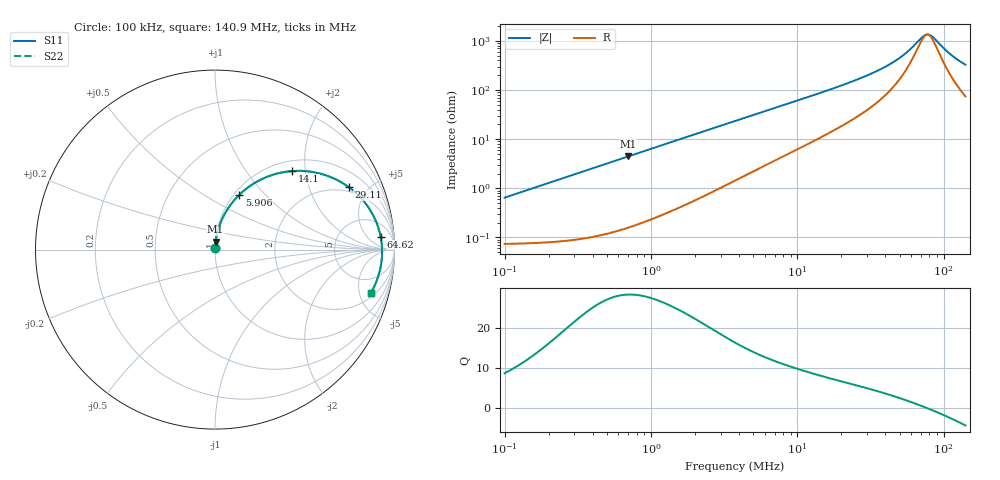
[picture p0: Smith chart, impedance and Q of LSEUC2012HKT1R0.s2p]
! LSEUC2012HKT1R0  S-PARAMETER MODEL  ( Standard Model )
! Model Generated by TAIYO YUDEN Corporation (http://www.ty-top.com)
! Version 1.0
! TAIYO YUDEN Control No. 20230502
! Copyright(c) 2023 TAIYO YUDEN CO.,LTD. All Rights Reserved.
! Product Description (link to TY-COMPAS)
! https://ds.yuden.co.jp/TYCOMPAS/or/detail?pn=LSEUC2012HKT1R0M&u=M
! Products Name : Inductors
! Characteristics :
!  Inductance : 1.0 [uH] , SRF(min) : - [Hz] , DC Resistance(max) : 0.078 [Ohm]
!  Rated Current : Saturation  3200 [mA] , Temp Rise  2300 [mA] (40 [degC])
!  Case Size : 2.0 x 1.2 / 0.079 x 0.047 [mm/inch] , Thickness : 0.8 / 0.031 [mm/inch]
!  (Conditions: Temperature = 25 [degC] , DC Bias Current = 0 [A])
! External Node Assignments :
!  1  o---GGG---o  2
! GND o---------o GND
! Frequency Range : 0.1MHz  -  140.89697MHz  [ 402 STEP ]
# MHz S RI R 50
! Freq[MHz].  S11 Real  S11 Imag  S21 Real  S21 Imag  S12 Real  S12 Imag  S22 Real  S22 Imag
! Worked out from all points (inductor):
!   401 points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, 100 kHz to 140.9 MHz, reference 50 ohm
!   read as one part in series: L = 1.02 uH near 103.7 kHz
!   highest Q = 28.2 at 695.6 kHz (marker M1), where L = 1.02 uH
!   self-resonance near 77.34 MHz
!   S11 on the Smith chart (normalised r, x): 100 kHz: 1.00, +0.01; 5.906 MHz: 1.06, +0.72; 14.1 MHz: 1.21, +1.70; 29.11 MHz: 1.73, +3.73; 64.62 MHz: 13, +13; 140.9 MHz: 2.48, -6.36
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0.1  0.00078 0.0064  0.9992 -0.0064  0.9992 -0.0064  0.00078 0.0064
0.336853  0.0014 0.0215  0.9986 -0.0215  0.9986 -0.0215  0.0014 0.0215
0.695555  0.00353 0.0441  0.9965 -0.0441  0.9965 -0.0441  0.00353 0.0441
1.134703  0.00781 0.0712  0.9922 -0.0712  0.9922 -0.0712  0.00781 0.0712
2.101545  0.0229 0.1283  0.9771 -0.1283  0.9771 -0.1283  0.0229 0.1283
3.753625  0.0636 0.2152  0.9364 -0.2152  0.9364 -0.2152  0.0636 0.2152
5.905507  0.1348 0.3046  0.8652 -0.3046  0.8652 -0.3046  0.1348 0.3046
8.641209  0.2373 0.3806  0.7627 -0.3806  0.7627 -0.3806  0.2373 0.3806
12.64421  0.3832 0.4318  0.6168 -0.4318  0.6168 -0.4318  0.3832 0.4318
14.09696  0.431 0.4377  0.569 -0.4377  0.569 -0.4377  0.431 0.4377
20.25678  0.5955 0.4209  0.4045 -0.4209  0.4045 -0.4209  0.5955 0.4209
29.10821  0.7442 0.3489  0.2558 -0.3489  0.2558 -0.3489  0.7442 0.3489
42.59248  0.8584 0.2297  0.1416 -0.2297  0.1416 -0.2297  0.8584 0.2297
52.94195  0.9001 0.1496  0.0999 -0.1496  0.0999 -0.1496  0.9001 0.1496
64.62413  0.9228 0.0719  0.0772 -0.0719  0.0772 -0.0719  0.9228 0.0719
73.36696  0.9296 0.0213  0.0704 -0.0213  0.0704 -0.0213  0.9296 0.0213
77.46709  0.9308 -0.000664  0.0692 0.000664  0.0692 0.000664  0.9308 -0.000664
80.32704  0.9309 -0.0153  0.0691 0.0153  0.0691 0.0153  0.9309 -0.0153
84.81615  0.9302 -0.0374  0.0698 0.0374  0.0698 0.0374  0.9302 -0.0374
111.3172  0.9097 -0.1481  0.0903 0.1481  0.0903 0.1481  0.9097 -0.1481
126.377  0.8899 -0.1991  0.1101 0.1991  0.1101 0.1991  0.8899 -0.1991
140.897  0.8674 -0.242  0.1326 0.242  0.1326 0.242  0.8674 -0.242
